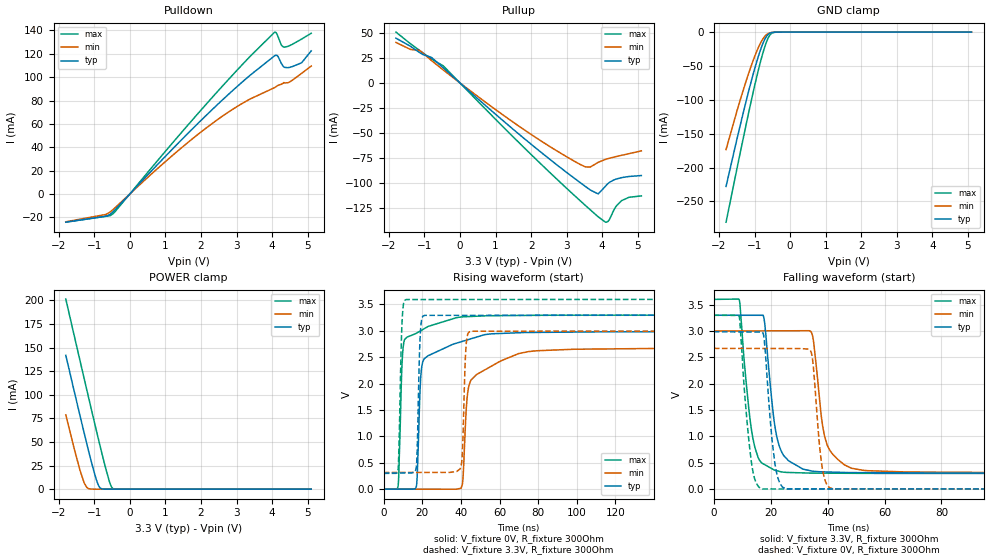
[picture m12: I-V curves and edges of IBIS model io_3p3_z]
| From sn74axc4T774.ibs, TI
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|   io_3p3_z Model
[Model]   io_3p3_z
Model_type   I/O
Polarity   Non-Inverting
Enable   Active-Low
Vinl = 0.8
Vinh = 2
Vmeas = 1.65
Vref = 0
Cref = 2pF
Rref = 100000
|   typ   min   max
C_comp   3.045pF   2.580pF   3.293pF
| Where Nom  PVT is Nominal Process, 3.3V, 27C
|   Fast PVT is Strong Process,  3.6V, -40C
|   Slow PVT is Weak Process,   3.0V, 130C
[Voltage Range]   3.3   3   3.6
|Junction Temperature
[Temperature Range]   27   130   -40
[Pullup Reference]   3.3   3   3.6
[Pulldown Reference]   0   -0   0
[Power Clamp Reference]   3.3   3   3.6
[GND Clamp Reference]   0   0   0
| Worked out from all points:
|   slope of the pulldown table from 0 to 0.495 V, typ, clamps not added: 30.7 ohm
|   slope of the pullup table from 0 to 0.495 V, typ, clamps not added: 31.8 ohm
|   GND clamp passes 1 mA (typ) near -0.54 V on its own axis
|   POWER clamp passes 1 mA (typ) near -0.83 V on its own axis
|   falling waveform, V_fixture 3.3V, R_fixture 300Ohm: 20-80 % time 3.91ns typ, 4.01ns min, 3.78ns max; typ from 3.3 V to 0.305 V
|   rising waveform, V_fixture 0V, R_fixture 300Ohm: 20-80 % time 2.39ns typ, 5.64ns min, 1.85ns max; typ from 0 V to 2.98 V
|   rising waveform, V_fixture 3.3V, R_fixture 300Ohm: 20-80 % time 1.2ns typ, 1.35ns min, 1.26ns max; typ from 0.305 V to 3.3 V
|   falling waveform, V_fixture 0V, R_fixture 300Ohm: 20-80 % time 2.83ns typ, 2.51ns min, 3.05ns max; typ from 2.98 V to 0 V
[Pulldown]
|   Voltage   I(typ)   I(min)   I(max)
-1.8V     -24.09mA   -23.8mA    -24.15mA
-675.3mV  -19.06mA   -17.55mA   -19.12mA
-475.2mV  -15.33mA   -13.45mA   -16.99mA
1.077V    34.65mA    29.76mA    39.28mA
2.236V    69.91mA    58.52mA    79.91mA
3.203V    96.93mA    78.23mA    112mA
4.072V    118.3mA    91.06mA    138.5mA
4.168V    117.6mA    93mA       134.6mA
4.258V    111.8mA    93.9mA     127.5mA
4.348V    108.5mA    95.11mA    125.7mA
4.831V    112.3mA    103.3mA    132.6mA
5.1V      122.5mA    109.5mA    137.6mA
[GND Clamp]
|   Voltage   I(typ)   I(min)   I(max)
-1.8V     -227.8mA   -173.4mA   -280.6mA
-1.372V   -131.2mA   -95.11mA   -170.7mA
-1.151V   -84.56mA   -58.82mA   -115.9mA
-944.4mV  -44.95mA   -29.29mA   -67.54mA
-813.3mV  -23.61mA   -14.42mA   -40.11mA
-709.8mV  -10.58mA   -6.214mA   -21.59mA
-606.3mV  -2.952mA   -1.889mA   -7.765mA
-516.6mV  -668.4uA   -524.4uA   -1.826mA
-406.2mV  -131.4uA   -108.9uA   -233.1uA
-68.1mV   -1.279uA   -1.561uA   -1.232uA
5.1V      0A         0A         0A
[Pullup]
|   Voltage   I(typ)   I(min)   I(max)
-1.8V     44.59mA    40.29mA    50.61mA
-1.131V   30.15mA    32.18mA    32.25mA
-468.3mV  14.94mA    12.9mA     16.97mA
1.581V    -48.73mA   -41.19mA   -56.73mA
3.299V    -97.16mA   -79.64mA   -114.7mA
3.658V    -106.5mA   -83.82mA   -126.2mA
3.879V    -110.4mA   -79.28mA   -133.1mA
4.086V    -103.1mA   -76.21mA   -138.6mA
4.162V    -100.2mA   -75.41mA   -137.9mA
4.389V    -95.8mA    -73.37mA   -122.8mA
4.548V    -94.32mA   -72.09mA   -117.2mA
5.1V      -92.27mA   -67.68mA   -112.5mA
[POWER Clamp]
|   Voltage   I(typ)   I(min)   I(max)
-1.8V     141.9mA    78.74mA    201.4mA
-1.565V   104.1mA    43.12mA    163mA
-1.407V   78.83mA    20.87mA    137.2mA
-1.296V   61.5mA     8.016mA    119.2mA
-1.214V   48.71mA    2.066mA    105.8mA
-985.8mV  15.65mA    4.518uA    69.3mA
-868.5mV  3.093mA    456.4nA    50.79mA
-771.9mV  146.4uA    317.2nA    35.85mA
-571.8mV  157.9nA    299.2nA    7.669mA
-516.6mV  99.8nA     296.5nA    2.383mA
-468.3mV  91.41nA    294nA      390.4uA
5.1V      0A         0A         0A
[Ramp]
R_load = 300
|   typ   min   max
dV/dt_r   1.79089/2.35615e-09   1.60246/5.29707e-09   1.97921/1.83668e-09
dV/dt_f   1.79679/3.89831e-09   1.61093/4.00667e-09   1.98108/3.77581e-09
[Falling Waveform]
V_fixture = 3.3V
V_fixture_min = 3V
V_fixture_max = 3.6V
R_fixture = 300Ohm
C_fixture = 0F
|   Time   V(typ)   V(min)   V(max)
0s        3.3V       3V         3.6V
8.946ns   3.299V     3.002V     3.596V
13.2ns    3.299V     3.002V     1.141V
17.36ns   3.299V     3.003V     481.5mV
21.1ns    1.338V     3.004V     367.9mV
23.77ns   716.3mV    3.004V     327.1mV
34.41ns   345.2mV    2.964V     304.3mV
39.79ns   326.6mV    848.4mV    303.2mV
52.53ns   313.3mV    357.9mV    300.4mV
500ns     305.4mV    315.1mV    298.2mV
[Rising Waveform]
V_fixture = 0V
V_fixture_min = 0V
V_fixture_max = 0V
R_fixture = 300Ohm
C_fixture = 0F
|   Time   V(typ)   V(min)   V(max)
0s        187.1nV    802.2nV    87.44nV
7.465ns   -200.5uV   -100.3uV   51.79mV
10.82ns   -290.8uV   -145.8uV   2.83V
17.04ns   75.94mV    -230uV     2.955V
20.29ns   2.416V     -274uV     3.024V
37.67ns   2.764V     -9.283uV   3.247V
40.79ns   2.799V     101.2mV    3.263V
45.14ns   2.847V     2.062V     3.27V
74.99ns   2.967V     2.605V     3.291V
500ns     2.985V     2.671V     3.299V
[Rising Waveform]
V_fixture = 3.3V
V_fixture_min = 3V
V_fixture_max = 3.6V
R_fixture = 300Ohm
C_fixture = 0F
|   Time   V(typ)   V(min)   V(max)
0s        305.4mV    315.1mV    298.2mV
7.408ns   306.7mV    315.6mV    357.9mV
9.528ns   307.1mV    315.8mV    3.165V
11.64ns   307.5mV    315.9mV    3.591V
16.93ns   428.6mV    316.3mV    3.591V
18.98ns   2.947V     316.5mV    3.591V
21.2ns    3.291V     316.6mV    3.591V
40.07ns   3.291V     434.1mV    3.591V
45.22ns   3.291V     2.991V     3.592V
500ns     3.3V       3V         3.6V
[Falling Waveform]
|Gnd
V_fixture = 0V
V_fixture_min = 0V
V_fixture_max = 0V
R_fixture = 300Ohm
C_fixture = 0F
|   Time   V(typ)   V(min)   V(max)
0s        2.985V     2.671V     3.299V
8.946ns   2.983V     2.67V      3.274V
13.2ns    2.982V     2.669V     519.5mV
17.15ns   2.968V     2.669V     3.903mV
21.51ns   479.2mV    2.668V     3.868mV
25.49ns   5.227mV    2.668V     3.836mV
34.26ns   5.131mV    2.594V     3.765mV
38.16ns   5.088mV    388.3mV    3.733mV
41.85ns   5.047mV    6.121mV    3.703mV
500ns     198.4nV    788.7nV    100.7nV
